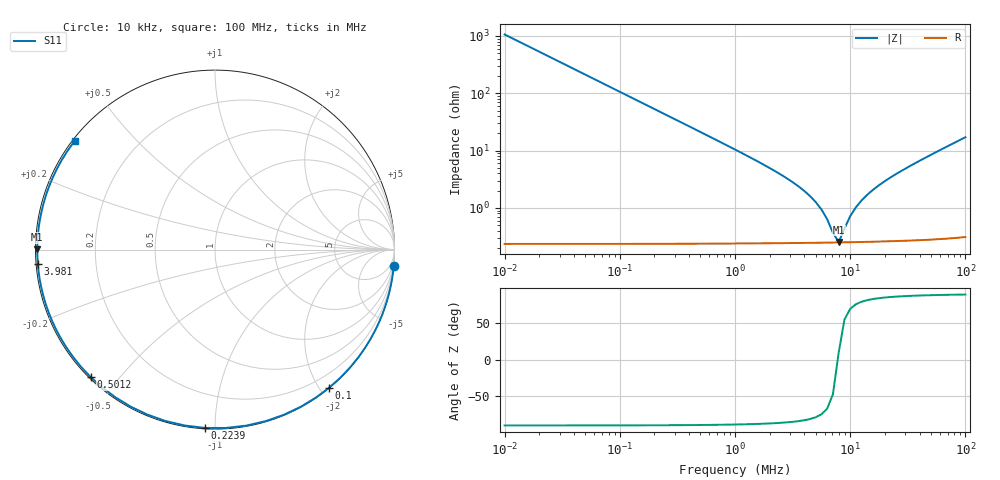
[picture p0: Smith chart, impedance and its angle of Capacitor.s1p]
! Touchstone file was created by TriD Version 2024.1.0 (64-bit) (06.06.2024)
! (C) EMCoS 1999-2024
! Project : D:\Demo\TRID_Capacitor_Capacitor\Capacitor.in
! Date  : 2024-09-16  13:13:36
# HZ S RI R  50.00
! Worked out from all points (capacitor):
!   81 points, 10 kHz to 100 MHz, reference 50 ohm
!   read as one part to ground: C = 15 nF near 10 kHz
!   lowest |Z| = 253 mohm at 7.943 MHz (marker M1)
!   series resonance near 7.828 MHz, so ESL is about 28 nH
!   S11 on the Smith chart (normalised r, x): 10 kHz: 0, -21; 100 kHz: 0.00, -2.12; 223.9 kHz: 0.00, -0.95; 501.2 kHz: 0.00, -0.42; 3.981 MHz: 0.00, -0.04; 100 MHz: 0.01, +0.34
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10000  0.9955 -0.094
17782.8  0.986 -0.1664
31622.8  0.9564 -0.2915
44668.4  0.9148 -0.403
63095.7  0.8369 -0.546
79432.8  0.7533 -0.6559
100000  0.6354 -0.77
125893  0.4779 -0.8756
158489  0.2825 -0.9557
199526  0.0606 -0.9937
223872  -0.0541 -0.9936
251189  -0.1672 -0.9803
316228  -0.378 -0.9188
398107  -0.5552 -0.8228
501187  -0.6925 -0.7102
707946  -0.8303 -0.5414
1000000  -0.9082 -0.3963
1778280  -0.9655 -0.2212
3162280  -0.9841 -0.1107
3981070  -0.9872 -0.078
7943280  -0.9901 0.00165
1e7  -0.9896 0.0266
1.99526e7  -0.983 0.1149
3.16228e7  -0.9689 0.2004
4.46684e7  -0.9462 0.2886
6.30957e7  -0.9026 0.4045
7.94328e7  -0.854 0.4988
1e8  -0.7819 0.6055
